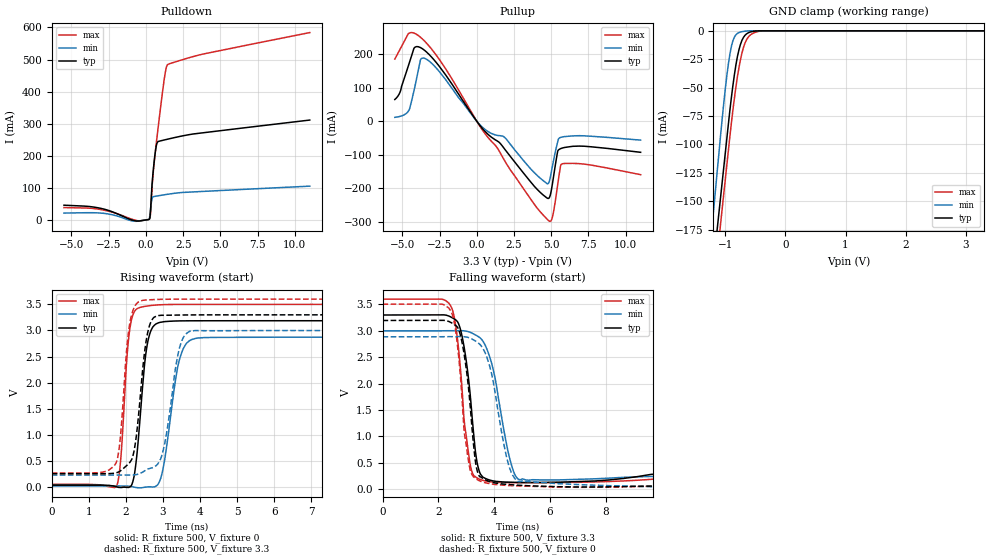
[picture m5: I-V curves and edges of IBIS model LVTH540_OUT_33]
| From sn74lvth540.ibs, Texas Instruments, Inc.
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[Model]   LVTH540_OUT_33
Model_type  3-state
Enable   Active-Low
Vref =   0
Rref =   500
Cref =   50p
Vmeas =   1.5
| variable   typ   min   max
C_comp   3.42pF   2.81pF   4.72pF
| C_pullup   4.02pF   0.55pF   5.35pF
| C_pulldown   8.39pF   1.77pF   34.76pF
| C_tri-state   3.42pF   2.81pF   4.72pF
[Temperature Range]   40   -40   100
| Ambient temperature   25   -40   85
[Voltage range]   3.3   3   3.6
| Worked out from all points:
|   slope of the pulldown table from 0 to 0.495 V, typ, clamps not added: 3.18 ohm
|   slope of the pullup table from 0 to 0.495 V, typ, clamps not added: 17.9 ohm
|   GND clamp passes 1 mA (typ) near -0.58 V on its own axis
|   rising waveform, R_fixture 500, V_fixture 0: 20-80 % time 235ps typ, 338ps min, 186ps max; typ from 0.041 V to 3.19 V
|   falling waveform, R_fixture 500, V_fixture 3.3: 20-80 % time 375ps typ, 593ps min, 352ps max; typ from 3.3 V to 0.26 V
|   rising waveform, R_fixture 500, V_fixture 3.3: 20-80 % time 264ps typ, 348ps min, 216ps max; typ from 0.261 V to 3.3 V
|   falling waveform, R_fixture 500, V_fixture 0: 20-80 % time 373ps typ, 602ps min, 357ps max; typ from 3.2 V to 0.041 V
[GND Clamp]
| LVTH540_OUT_33
|   Voltage   I(typ)   I(min)   I(max)
-5.5V     -2.861A    -3.034A    -2.892A
-1.24V    -226.4mA   -182.9mA   -251mA
-1.21V    -211.3mA   -165.7mA   -235.5mA
-1.17V    -191.4mA   -142.9mA   -215.1mA
-1.075V   -144mA     -89.19mA   -167.4mA
-975mV    -94.37mA   -39.09mA   -117.7mA
-925mV    -69.94mA   -20.46mA   -92.96mA
-875mV    -48.14mA   -8.719mA   -69.85mA
-800mV    -22.75mA   -2.299mA   -40.47mA
-725mV    -8.466mA   -746.4uA   -19.69mA
-575mV    -873.9uA   -11.47uA   -3.26mA
3.3V      32.83pA    25.31pA    1.688nA
[Pulldown]
| LVTH540_OUT_33
|   Voltage   I(typ)   I(min)   I(max)
-5.5V     45.71mA    21.15mA    38.31mA
-3.03V    35.84mA    21.15mA    32.09mA
-705mV    -3.067mA   -4.477mA   -1.231mA
215mV     1.677mA    2.589mA    1.896mA
305mV     26.06mA    31.6mA     17.21mA
425mV     118.9mA    68.07mA    110mA
580mV     192.7mA    73.06mA    190.3mA
710mV     233.6mA    74.11mA    244.7mA
1.225V    249.1mA    78.08mA    437.1mA
1.445V    251.5mA    79.68mA    483.5mA
3.79V     271.3mA    88.58mA    516.6mA
11V       311.3mA    105.1mA    584.1mA
[Pullup]
| LVTH540_OUT_33
|   Voltage   I(typ)   I(min)   I(max)
-5.5V     64.85mA    11.59mA    185.8mA
-4.55V    171.3mA    33.05mA    262.9mA
-4.2V     218.9mA    93.95mA    263.1mA
-3.78V    220mA      183.2mA    250.9mA
-3.47V    210.5mA    187.4mA    237.9mA
285mV     -16.78mA   -13.82mA   -20.22mA
1.85V     -81.89mA   -47.23mA   -116.3mA
4.875V    -228mA     -179.2mA   -298.5mA
5.105V    -179.8mA   -128.5mA   -281.7mA
5.43V     -90.52mA   -62.02mA   -190.5mA
5.695V    -80.75mA   -47.47mA   -128mA
11V       -92.87mA   -56.45mA   -159.6mA
[Ramp]
| LVTH540_OUT_33
| variable   typ   min   max
dV/dt_r   1.91/2.42E-10   1.73/3.49E-10   2.10/1.91E-10
dV/dt_f   1.91/3.88E-10   1.70/6.09E-10   2.09/3.76E-10
R_load = 500
[Rising Waveform]
| LVTH540_OUT_33
R_fixture =   500
C_fixture =   0
L_fixture =   0
V_fixture =   0
V_fixture_min = 0
V_fixture_max = 0
|   Time   V(typ)   V(min)   V(max)
0s        41.42mV    24.68mV    57.22mV
1.745ns   11.01mV    25.42mV    17.21mV
1.855ns   -3.563mV   25.36mV    488.8mV
2.145ns   28.38mV    14.06mV    3.186V
2.54ns    2.564V     4.468mV    3.464V
2.73ns    3.071V     6.205mV    3.482V
2.995ns   3.165V     330.6mV    3.494V
3.46ns    3.184V     2.481V     3.499V
3.945ns   3.186V     2.856V     3.499V
50ns      3.188V     2.873V     3.5V
[Falling Waveform]
| LVTH540_OUT_33
R_fixture =   500
C_fixture =   0
L_fixture =   0
V_fixture =   3.3
V_fixture_min = 3
V_fixture_max = 3.6
|   Time   V(typ)   V(min)   V(max)
0s        3.3V       3V         3.6V
2.425ns   3.269V     3.002V     3.488V
2.62ns    3.209V     3.002V     3.104V
2.815ns   2.979V     3.004V     2.138V
3.165ns   1.655V     2.967V     408.6mV
3.415ns   439.2mV    2.897V     204.9mV
3.835ns   172.8mV    2.516V     142.1mV
4.54ns    132.6mV    618.8mV    123.4mV
4.92ns    127.3mV    178.2mV    122.3mV
50ns      260.2mV    234.4mV    273mV
[Rising Waveform]
| LVTH540_OUT_33
R_fixture =   500
C_fixture =   0
L_fixture =   0
V_fixture =   3.3
V_fixture_min = 3
V_fixture_max = 3.6
|   Time   V(typ)   V(min)   V(max)
0s        260.8mV    234.8mV    273.4mV
1.725ns   275.2mV    234.6mV    451.6mV
1.845ns   310.7mV    234.4mV    910.9mV
2.11ns    480.5mV    234.2mV    3.156V
2.27ns    916.7mV    240.9mV    3.498V
2.48ns    2.438V     303mV      3.579V
2.94ns    3.29V      547.8mV    3.596V
3.445ns   3.296V     2.664V     3.599V
3.86ns    3.298V     2.998V     3.6V
50ns      3.3V       3V         3.6V
[Falling Waveform]
| LVTH540_OUT_33
R_fixture =   500
C_fixture =   0
L_fixture =   0
V_fixture =   0
V_fixture_min = 0
V_fixture_max = 0
|   Time   V(typ)   V(min)   V(max)
0s        3.196V     2.888V     3.505V
2.415ns   3.168V     2.89V      3.401V
2.8ns     2.898V     2.892V     2.086V
2.93ns    2.54V      2.888V     1.087V
3.135ns   1.613V     2.862V     378.2mV
3.395ns   344.6mV    2.784V     181mV
3.955ns   127mV      2.069V     94.21mV
4.47ns    90.52mV    553.2mV    70.95mV
4.9ns     73.94mV    139.4mV    61.74mV
50ns      41.43mV    24.68mV    57.3mV
